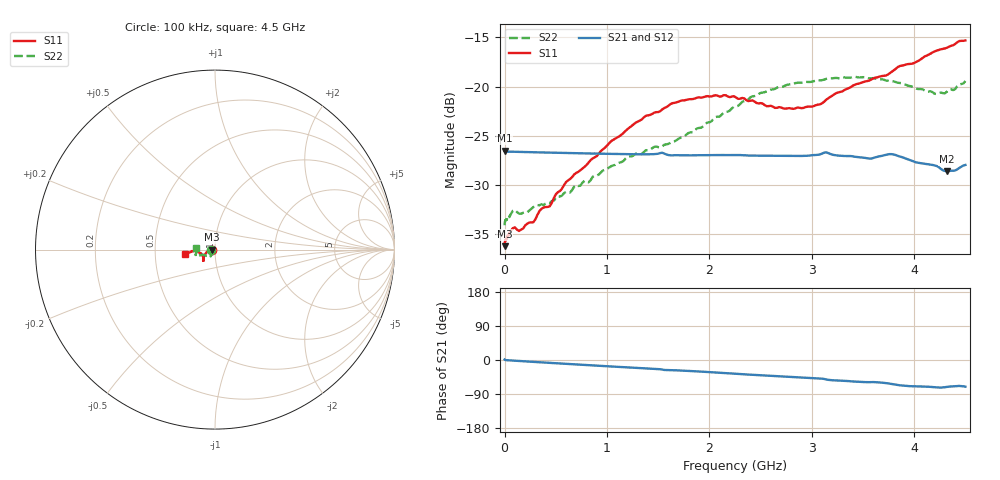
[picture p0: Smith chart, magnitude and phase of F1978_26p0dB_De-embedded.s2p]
! Integrated Device Technology
! Corporate Headquarters
! 6024 Silver Creek Valley Road
! San Jose, CA 95138  USA
! Phone:  1-408-284-8200
! Toll Free:  1-800-223-1366
! Webpage:  http://www.idt.com/
! Timing and RF Division
! 515 Groton Road, Suite 102
! Westford, MA 01886-6024
! Device:  F1978
! Description: 6-bit, 75 ohm, 0.5 dB Digital Step Attenuator
! Frequency:  5.0 MHz -  3.00 GHz
! Package:  4x4 mm QFN Plastic Package: 20 pin
! Ports:  2 RF, 11 DC
!  Pin  1  = D5 (16 dB)
!  Pin  2  = RF1  =  Port 1
!  Pin  3  = Serial Data In (DATA)
!  Pin  4  = Serial Clock (CLK)
!  Pin  5  = Serial Latch Enable (LE)
!  Pin  6  = VDD
!  Pin  7  = NC
!  Pin  8  = NC
!  Pin  9  = NC
!  Pin 10  = GND
!  Pin 11  = GND
!  Pin 12  = NC
!  Pin 13  = VMODE
!  Pin 14  = RF2  =  Port 2
!  Pin 15  = D4 (8 dB)
!  Pin 16  = D3 (4 dB)
!  Pin 17  = D2 (2 dB)
!  Pin 18  = NC
!  Pin 19  = D1 (1 dB)
!  Pin 20  = D0 (0.5 dB)
! State:  52
! Atten State:  26.0 dB
! Voltage:  +3.30 Volts
! Current:  0.591 mA
! Data:  The device was measured on a F1975 evaluation board which has
!  individual transmission lines to the RF pins.  Data was collected
!  using a calibrated network analyzer.  The evaluation board was
!  de-embedded using Automatic Fixture Removal (AFR).
!  The reference plane is the edge of the package pin.
! Misc:
!  Action Tracker AT0416
! Date Measured:  2018-02-08
! Date:  2018-03-26  MJV
! Note:
!  Integrated Device Technology supplies this data as a sample of measured
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# GHz S dB R 75
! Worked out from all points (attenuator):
!   291 points, 100 kHz to 4.5 GHz, reference 75 ohm
!   highest |S21| = -26.53 dB at 300 kHz (marker M1); lowest = -28.6 dB at 4.32 GHz (marker M2)
!   lowest |S11| = -36.2 dB at 100 kHz (marker M3), VSWR 1.03, Z = 72.7 - j1.26e-05 ohm
!   |S11| at or under -10 dB: start of sweep to end of sweep
!   |S22| runs from -34.1 to -19.0 dB; largest |S21 - S12| = 0.00016
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0.0001  -36.22 -180.0  -26.53 1.2  -26.56 1.2  -34.10 -179.1
0.0003  -36.10 -179.3  -26.53 1.1  -26.55 1.1  -34.01 -178.6
0.011  -35.54 -178.1  -26.61 -0.3  -26.61 -0.3  -33.55 -176.5
0.08  -34.39 -176.5  -26.62 -1.5  -26.62 -1.5  -32.63 -169.3
0.14  -34.68 -175.8  -26.64 -2.6  -26.64 -2.6  -32.90 -160.5
0.28  -33.79 -179.9  -26.67 -4.9  -26.67 -4.9  -32.25 -151.0
0.36  -32.43 180.0  -26.70 -6.2  -26.69 -6.2  -31.96 -143.4
0.44  -32.18 -179.4  -26.71 -7.5  -26.71 -7.5  -31.86 -137.6
0.6  -29.71 -175.8  -26.76 -10.1  -26.75 -10.1  -30.70 -131.8
0.76  -28.35 -169.1  -26.79 -12.6  -26.78 -12.7  -29.77 -128.2
1.28  -23.67 -152.7  -26.88 -20.7  -26.88 -20.7  -26.82 -123.8
1.52  -22.50 -145.4  -26.76 -24.3  -26.75 -24.3  -26.18 -130.5
1.64  -21.69 -142.7  -26.99 -26.8  -26.99 -26.8  -25.62 -134.6
1.88  -21.13 -138.7  -26.98 -30.1  -26.98 -30.1  -24.25 -146.6
2.26  -21.11 -137.1  -26.96 -36.3  -26.96 -36.3  -22.00 -157.5
2.64  -22.17 -147.5  -27.03 -42.4  -27.03 -42.4  -20.24 -159.1
3.02  -21.98 -164.2  -26.96 -48.0  -26.96 -48.1  -19.46 -159.9
3.42  -19.81 -175.6  -27.13 -57.0  -27.13 -57.0  -19.00 -164.2
3.76  -18.66 -175.8  -26.87 -62.5  -26.87 -62.5  -19.43 -169.6
4.2  -16.43 -172.6  -28.02 -71.7  -28.02 -71.7  -20.74 178.9
4.32  -16.05 -172.1  -28.62 -70.9  -28.61 -70.9  -20.52 176.7
4.5  -15.31 -171.9  -27.97 -70.3  -27.96 -70.4  -19.44 174.0
